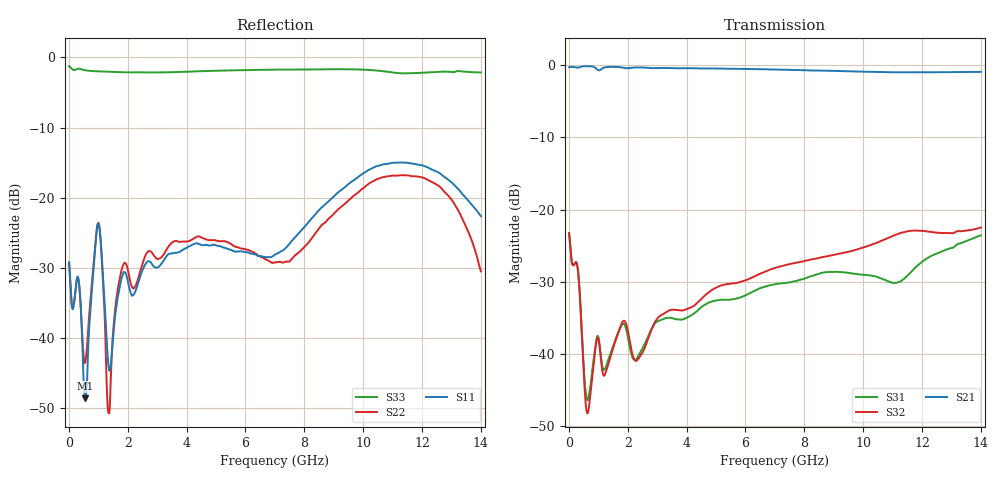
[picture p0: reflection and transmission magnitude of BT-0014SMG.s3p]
! MARKI MICROWAVE INC.
! Email:  info@markimicrowave.com  Phone:  408-778-4200
! Model Number:  BT-0014SM  Date:  12/12
! Filename:		BT_0014SM.S3P  Version: 1.0
! Description:  3-port S-parameter data for Bias Tee BT-0014SM
! Frequency Range: 	10 MHz to 14 GHz
! Port Configuration:	PORT 1: RF & DC
!  PORT 2: RF
!  Port 3: DC
! S3P File: Measurements: Mag<S11> Ang<S11> Mag<S12> Ang<S12> Mag<S13> Ang<S13> ! row 1
!  Mag<S21> Ang<S21> Mag<S22> Ang<S22> Mag<S23> Ang<S23> ! row 2
!  Mag<S31> Ang<S31> Mag<S32> Ang<S32> Mag<S33> Ang<S33> ! row 3
# Hz S  dB  R 50
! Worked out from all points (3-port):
!   801 points, 10 MHz to 14 GHz, reference 50 ohm
!   strongest paths, dB at 10 MHz, 3.507 GHz, 7.005 GHz, 10.5 GHz, 14 GHz:
!     S21: -0.2, -0.4, -0.6, -0.9, -0.9
!     S32: -23.3, -33.9, -28.1, -24.5, -22.5
!     S31: -23.3, -35.1, -30.4, -29.4, -23.6
!   lowest |S11| = -48.6 dB at 552.1 MHz (marker M1), VSWR 1.01, Z = 50.4 - j0.0941 ohm
!   |S11| at or under -10 dB: start of sweep to end of sweep
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1e7  -29.18 139.2  -0.25 -0.1  -23.27 -39.4
     -0.24 -0.4  -29.39 136.8  -23.38 -39.8
     -23.29 -39.0  -23.28 -38.9  -1.26 1.5
5.521125e8  -48.57 -14.5  -0.10 -26.3  -44.42 -91.9
            -0.10 -26.3  -43.55 -15.1  -45.78 -97.5
            -44.54 -92.8  -45.89 -98.6  -1.85 -33.3
9.893e8  -23.77 154.4  -0.64 -48.5  -37.54 -47.5
         -0.63 -48.4  -23.61 169.2  -37.83 -41.7
         -37.55 -46.9  -37.80 -41.9  -2.00 -57.6
1.356538e9  -44.18 110.8  -0.21 -63.9  -40.80 -38.4
            -0.20 -63.9  -50.71 -44.4  -41.28 -29.9
            -40.65 -38.1  -41.20 -29.6  -2.05 -78.2
1.846188e9  -30.75 138.0  -0.32 -88.3  -35.84 -68.9
            -0.31 -88.3  -29.60 176.0  -35.52 -57.7
            -35.86 -69.1  -35.49 -58.1  -2.14 -105.7
3.7873e9  -27.66 60.4  -0.40 -179.5  -35.29 -134.5
          -0.39 -179.5  -26.28 88.6  -33.98 -122.1
          -35.27 -134.4  -33.98 -122.1  -2.09 148.0
7.005e9  -28.10 -56.8  -0.56 28.1  -30.43 79.9
         -0.57 28.0  -29.22 -44.3  -28.14 92.6
         -30.37 79.9  -28.11 92.8  -1.75 -21.1
1.001285e10  -16.51 170.4  -0.85 -113.2  -29.13 -71.3
             -0.86 -113.4  -18.61 156.7  -25.33 -51.9
             -29.04 -71.0  -25.25 -51.8  -1.76 -179.1
1.179658e10  -15.24 90.2  -0.94 163.7  -28.09 -133.9
             -0.96 163.6  -16.95 70.7  -22.99 -146.8
             -27.96 -133.8  -22.92 -146.8  -2.25 98.4
1.4e10  -22.64 26.1  -0.87 61.0  -23.66 111.5
        -0.89 60.9  -30.48 -54.1  -22.59 109.6
        -23.59 111.6  -22.50 109.5  -2.16 -5.9
